(* Logix 5000 DataType export SD_State; software revision 20.01 *)

TYPE SD_State :   // smart drive状态数据
STRUCT
   Trip : BOOL;   // Trip bit位：0：正常，1：故障，触发条件是通过380V的开关进行触发产生
   WarningPresent : BOOL;   // Reserved
   RunningFWD : BOOL;   // 电机正向运行
   RunningRVS : BOOL;   // 电机反向运行
   Ready : BOOL;   // Ready bit位：0：故障，1：正常，触发条件系统各个子系统有异常就触发
   NetCtrlStat : BOOL;   // Reserved
   NetRefStats : BOOL;   // Reserved
   CurntFlow : BOOL;   // Reserved
   ReservedBit8 : BOOL;   // Reserved
   ReservedBit9 : BOOL;   // Reserved
   ReservedBit10 : BOOL;   // Reserved
   ReservedBit11 : BOOL;   // Reserved
   KeyPadOn : BOOL;   // Keypad On
   DiscOn : BOOL;   // Disconnecter On, 正常状态为ON(=1) 380V bit0相反
   ReservedBit14 : BOOL;   // Reserved
   ReservedBit15 : BOOL;   // Reserved
   ShortCircuit : BOOL;   // 短路
   OverLoad : BOOL;   // 过载
   PhaseLoss : BOOL;   // 缺相
   ReservedBit19 : BOOL;   // Reserved
   ReservedBit20 : BOOL;   // Reserved
   ControlPowerLost : BOOL;   // 控制电丢失
   ComFault : BOOL;   // 通讯错误
   ReservedBit23 : BOOL;   // Reserved
   PhaseImbalance : BOOL;   // 相位失衡
   ReservedBit25 : BOOL;   // Reserved
   ReservedBit26 : BOOL;   // Reserved
   ReservedBit27 : BOOL;   // Reserved
   ReservedBit28 : BOOL;   // Reserved
   HardwareFault : BOOL;   // 硬件故障
   ReservedBit30 : BOOL;   // Reserved
   ReservedBit31 : BOOL;   // Reserved
   Current : INT;   // 电流整数，需乘以0.01
   Input1 : BOOL;   // 输入1
   Input2 : BOOL;   // 输入2
   Input3 : BOOL;   // 输入3
   Input4 : BOOL;   // 输入4
   Input5 : BOOL;   // 输入5
   Input6 : BOOL;   // 输入6
   Input7 : BOOL;   // 输入7
   Input8 : BOOL;   // 输入8
END_STRUCT
END_TYPE
